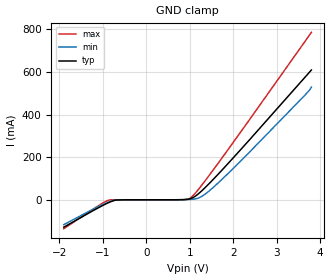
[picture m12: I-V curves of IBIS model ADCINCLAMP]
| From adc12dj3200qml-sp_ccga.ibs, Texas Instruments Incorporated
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[Model]   ADCINCLAMP
Model_type   Terminator
|   typ   min   max
C_comp   0.46pF   0.45pF   0.47pF
[Voltage Range]   1.9   1.8   2
[Temperature Range]   25   125   -40
[Power Clamp Reference]   1.9   1.8   2
[GND Clamp Reference]   0   0   0
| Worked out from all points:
|   GND clamp passes 1 mA (typ) near -0.65 V on its own axis
[GND Clamp]
|   Voltage   I(typ)   I(min)   I(max)
-1.9V     -128.7mA   -116.8mA   -135.6mA
-1.193V   -47.41mA   -40.93mA   -39.73mA
-856.9mV  -12.35mA   -9.69mA    -1.292mA
-691.6mV  -1.203mA   -830.6uA   -2.517uA
864.5mV   885.3uA    453.1uA    112.7uA
1.018V    5.206mA    1.701mA    8.834mA
1.132V    17.36mA    4.252mA    32.09mA
1.286V    43.74mA    17.05mA    70.98mA
1.685V    126.8mA    84.91mA    180.3mA
2.386V    283.8mA    225.8mA    379mA
3.675V    580mA      495.8mA    749.3mA
3.8V      609mA      528.8mA    785.6mA
